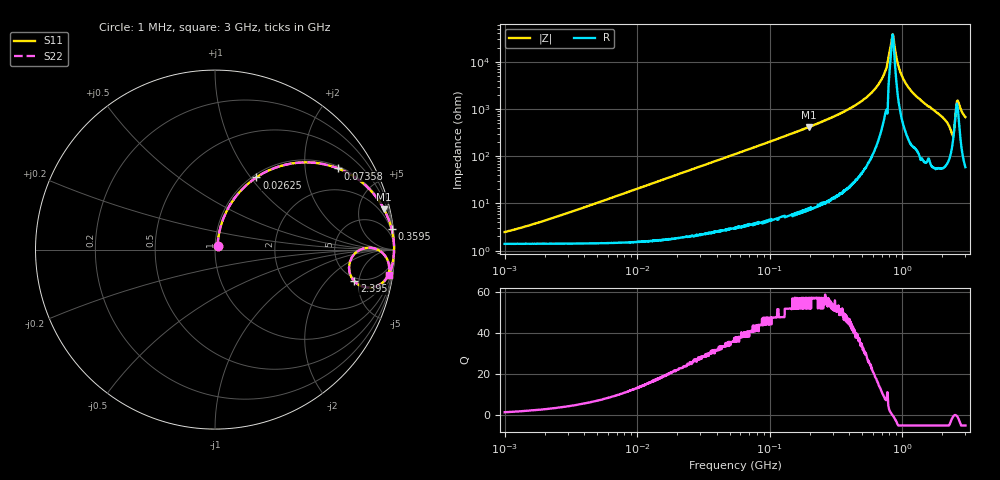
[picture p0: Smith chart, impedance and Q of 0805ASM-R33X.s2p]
!s-Parameter Generated by FASTRON Sdn. Bhd.
!FASTRON P/N : 0805ASM-R33X
!Keysight Technologies: E4991B_MY54100416_A.01.15
!Date: Fri Jun 19 14:52:23 2026
!Version  :Rev00  Fri Jun 19 14:52:23 2026
!Data & Calibration Information:
!Freq  S11  S21  S12  S22
!PortZ  Port1:50+j0  Port2:50+j0
!When reading reference impedance value at option line is always used.
! Remarks : This data is being provided solely for informational purposes.
# Hz S dB R 50
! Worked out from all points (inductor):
!   1601 points, 1 MHz to 3 GHz, reference 50 ohm
!   read as one part in series: L = 326 nH near 2.066 MHz
!   highest Q = 57.3 at 198.2 MHz (marker M1), where L = 336 nH
!   self-resonance near 845.9 MHz
!   S11 on the Smith chart (normalised r, x): 1 MHz: 1.03, +0.04; 26.25 MHz: 1.04, +1.07; 73.58 MHz: 1.07, +2.98; 359.5 MHz: 1, +17; 2.395 GHz: 4.51, -4.35; 3 GHz: 2, -13
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1000000  -32.20 54.6  -0.12 -1.2  -0.12 -1.2  -32.20 54.6
3804036  -22.20 75.3  -0.15 -4.4  -0.15 -4.4  -22.20 75.3
1.447069e7  -11.10 70.6  -0.49 -16.2  -0.49 -16.2  -11.10 70.6
2.624824e7  -6.68 60.2  -1.23 -27.6  -1.23 -27.6  -6.68 60.2
5.504702e7  -2.68 41.2  -3.62 -47.2  -3.62 -47.2  -2.68 41.2
7.358334e7  -1.71 33.4  -5.17 -55.2  -5.17 -55.2  -1.71 33.4
1.981861e8  -0.28 13.4  -12.70 -75.5  -12.70 -75.5  -0.28 13.4
2.083556e8  -0.25 12.7  -13.10 -76.3  -13.10 -76.3  -0.25 12.7
3.594878e8  -0.08 6.6  -18.80 -82.3  -18.80 -82.3  -0.08 6.6
6.296259e8  -0.02 2.1  -28.80 -84.8  -28.80 -84.8  -0.02 2.1
7.352784e8  -0.02 1.0  -35.20 -82.3  -35.20 -82.3  -0.02 1.0
7.925923e8  -0.02 0.4  -42.60 -73.2  -42.60 -73.2  -0.02 0.4
8.291033e8  -0.02 0.1  -48.50 -43.3  -48.50 -43.3  -0.02 0.1
8.543737e8  -0.02 -0.0  -51.30 18.5  -51.30 18.5  -0.02 -0.0
9.585869e8  -0.02 -0.9  -36.40 80.2  -36.40 80.2  -0.02 -0.9
1.097256e9  -0.03 -1.9  -29.80 83.5  -29.80 83.5  -0.03 -1.9
2.050964e9  -0.22 -8.8  -16.30 76.1  -16.30 76.1  -0.22 -8.8
2.301132e9  -0.78 -13.1  -12.60 62.0  -12.60 62.0  -0.78 -13.1
2.39512e9  -1.98 -12.8  -10.90 38.2  -10.90 38.2  -1.98 -12.8
2.51802e9  -1.20 0.6  -17.80 -4.4  -17.80 -4.4  -1.20 0.6
2.634014e9  -0.39 -2.8  -23.80 46.5  -23.80 46.5  -0.39 -2.8
3e9  -0.20 -8.3  -16.80 76.7  -16.80 76.7  -0.20 -8.3
